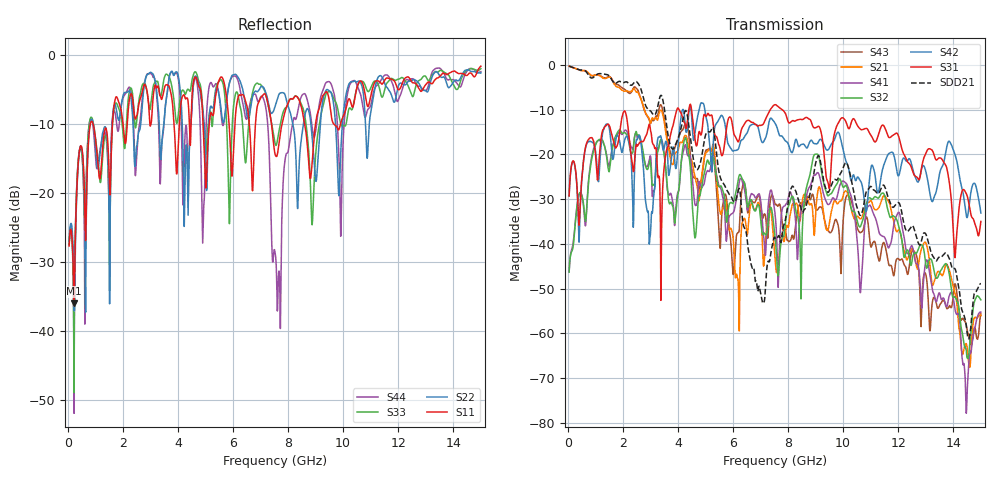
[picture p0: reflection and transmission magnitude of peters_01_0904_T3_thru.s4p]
# MHZ S RI R 50.00
! FREQ  S11  S12  S13  S14
!  S21  S22  S23  S24
!  S31  S32  S33  S34
!  S41  S42  S43  S44
!  REAL  IMAG  REAL  IMAG  REAL  IMAG  REAL  IMAG
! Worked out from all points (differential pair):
!   1496 points, 50 MHz to 15 GHz, reference 50 ohm
!   strongest paths, dB at 50 MHz, 3.79 GHz, 7.53 GHz, 11.27 GHz, 15 GHz:
!     S31: -29.3, -14.1, -8.9, -15.8, -35.0
!     S42: -29.3, -19.7, -13.1, -28.5, -33.1
!     S32: -46.3, -31.2, -38.5, -29.8, -52.5
!     S41: -46.2, -29.9, -33.5, -36.5, -55.2
!     S21: -0.3, -22.2, -43.4, -32.0, -56.0
!     S43: -0.3, -20.1, -31.1, -43.0, -55.6
!   taken as a pair (ports 1,3 in; 2,4 out), SDD21 dB: -0.2, -18.7, -38.8, -28.7, -48.9
!   lowest |S11| = -35.9 dB at 230 MHz (marker M1), VSWR 1.03, Z = 51.6 + j0.158 ohm
!   |S11| at or under -10 dB: start of sweep to 819.4 MHz; 922.9 MHz to 1.623 GHz (699.7 MHz wide, 55 % of centre); 7.398 GHz to 7.78 GHz (382.1 MHz wide, 5.04 % of centre)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
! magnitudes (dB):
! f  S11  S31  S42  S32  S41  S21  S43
! 50 MHz  -27.6  -29.3  -29.3  -46.3  -46.2  -0.3  -0.3
! 230 MHz  -35.9  -21.7  -21.8  -38.6  -37.9  -0.6  -0.6
! 5.27 GHz  -8.8  -12.6  -19.3  -20.0  -20.1  -17.7  -19.4
! 6.17 GHz  -6.4  -17.1  -18.9  -26.4  -28.6  -47.7  -37.5
! 7.66 GHz  -13.1  -9.4  -15.3  -46.1  -46.1  -43.9  -31.3
! 9.03 GHz  -9.1  -14.0  -17.6  -19.9  -24.3  -30.7  -32.4
! 15 GHz  -1.6  -35.0  -33.1  -52.5  -55.2  -56.0  -55.6
